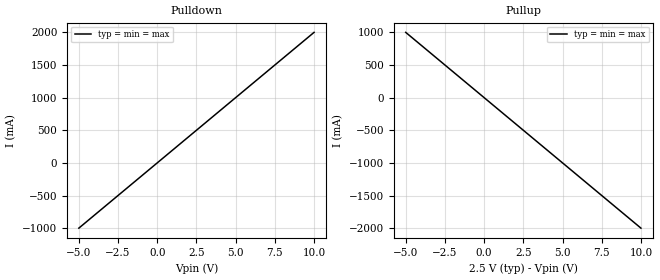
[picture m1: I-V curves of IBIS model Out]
[IBIS Ver]   3.2
[Comment Char]  |_char
[File Name]   bug40.ibs
[File Rev]   1.0
[Date]   May 3, 2000
[Component]   Test
[Manufacturer]   Test File
[Package]
| variable   typ   min   max
R_pkg   0.0m   NA   NA
L_pkg   0.0nH   NA   NA
C_pkg   0.0pF   NA   NA
[Pin]   signal_name   model_name   R_pin   L_pin   C_pin
  1   PAD   Term   NA   NA   NA
  2   PADN   Term   NA   NA   NA
  3   PAD   NC   NA   NA   NA
  4   PADN   NC   NA   NA   NA
| The pins below cause the incorrect error message:
  5   PAD   In   NA   NA   NA
  6   PADN   In   NA   NA   NA
  7   PAD   Out   NA   NA   NA
  8   PADN   Out   NA   NA   NA
[Series Pin Mapping]  pin_2   model_name   function_table_group
   1   2   Rseries
   3   4   Rseries
   5   6   Rseries
   7   8   Rseries
|   MODEL Rseries
[Model]   Rseries
Model_type   Series
C_comp   0.02pF   0.01pF  0.03pF
[Voltage Range]   2.50   2.30   2.70
| variable   R(typ)   R(min)   R(max)
[R Series]   100ohm   90ohm   110ohm
|   MODEL Term
[Model]   Term
Model_type   Terminator
Vinl  = 1.25V
Vinh = 2.5
C_comp   0.02pF   0.01pF  0.03pF
[Voltage Range]   2.50   2.30   2.70
|   MODEL In
[Model]   In
Model_type   Input
Vinl  = 1.25V
Vinh = 2.5
C_comp   0.02pF   0.01pF  0.03pF
[Voltage Range]   2.50   2.30   2.70
| Models and submodels in the file (4): Rseries (Series), Term (Terminator), In (Input), Out (Output)
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|   MODEL Out
[Model]   Out
Model_type   Output
Vmeas  = 1.25V
C_comp   0.02pF   0.01pF  0.03pF
[Voltage Range]   2.50   2.30   2.70
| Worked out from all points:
|   slope of the pulldown table from 0 to 0.375 V, typ, clamps not added: 5 ohm
|   slope of the pullup table from 0 to 0.375 V, typ, clamps not added: 5 ohm
[Pulldown]
-5V       -1A        -1A        -1A
10V       2A         2A         2A
[Pullup]
-5V       1A         1A         1A
10V       -2A        -2A        -2A
[Ramp]
dV/dt_r  1/1n 1/1n 1/1n
dV/dt_f  1/1n 1/1n 1/1n
